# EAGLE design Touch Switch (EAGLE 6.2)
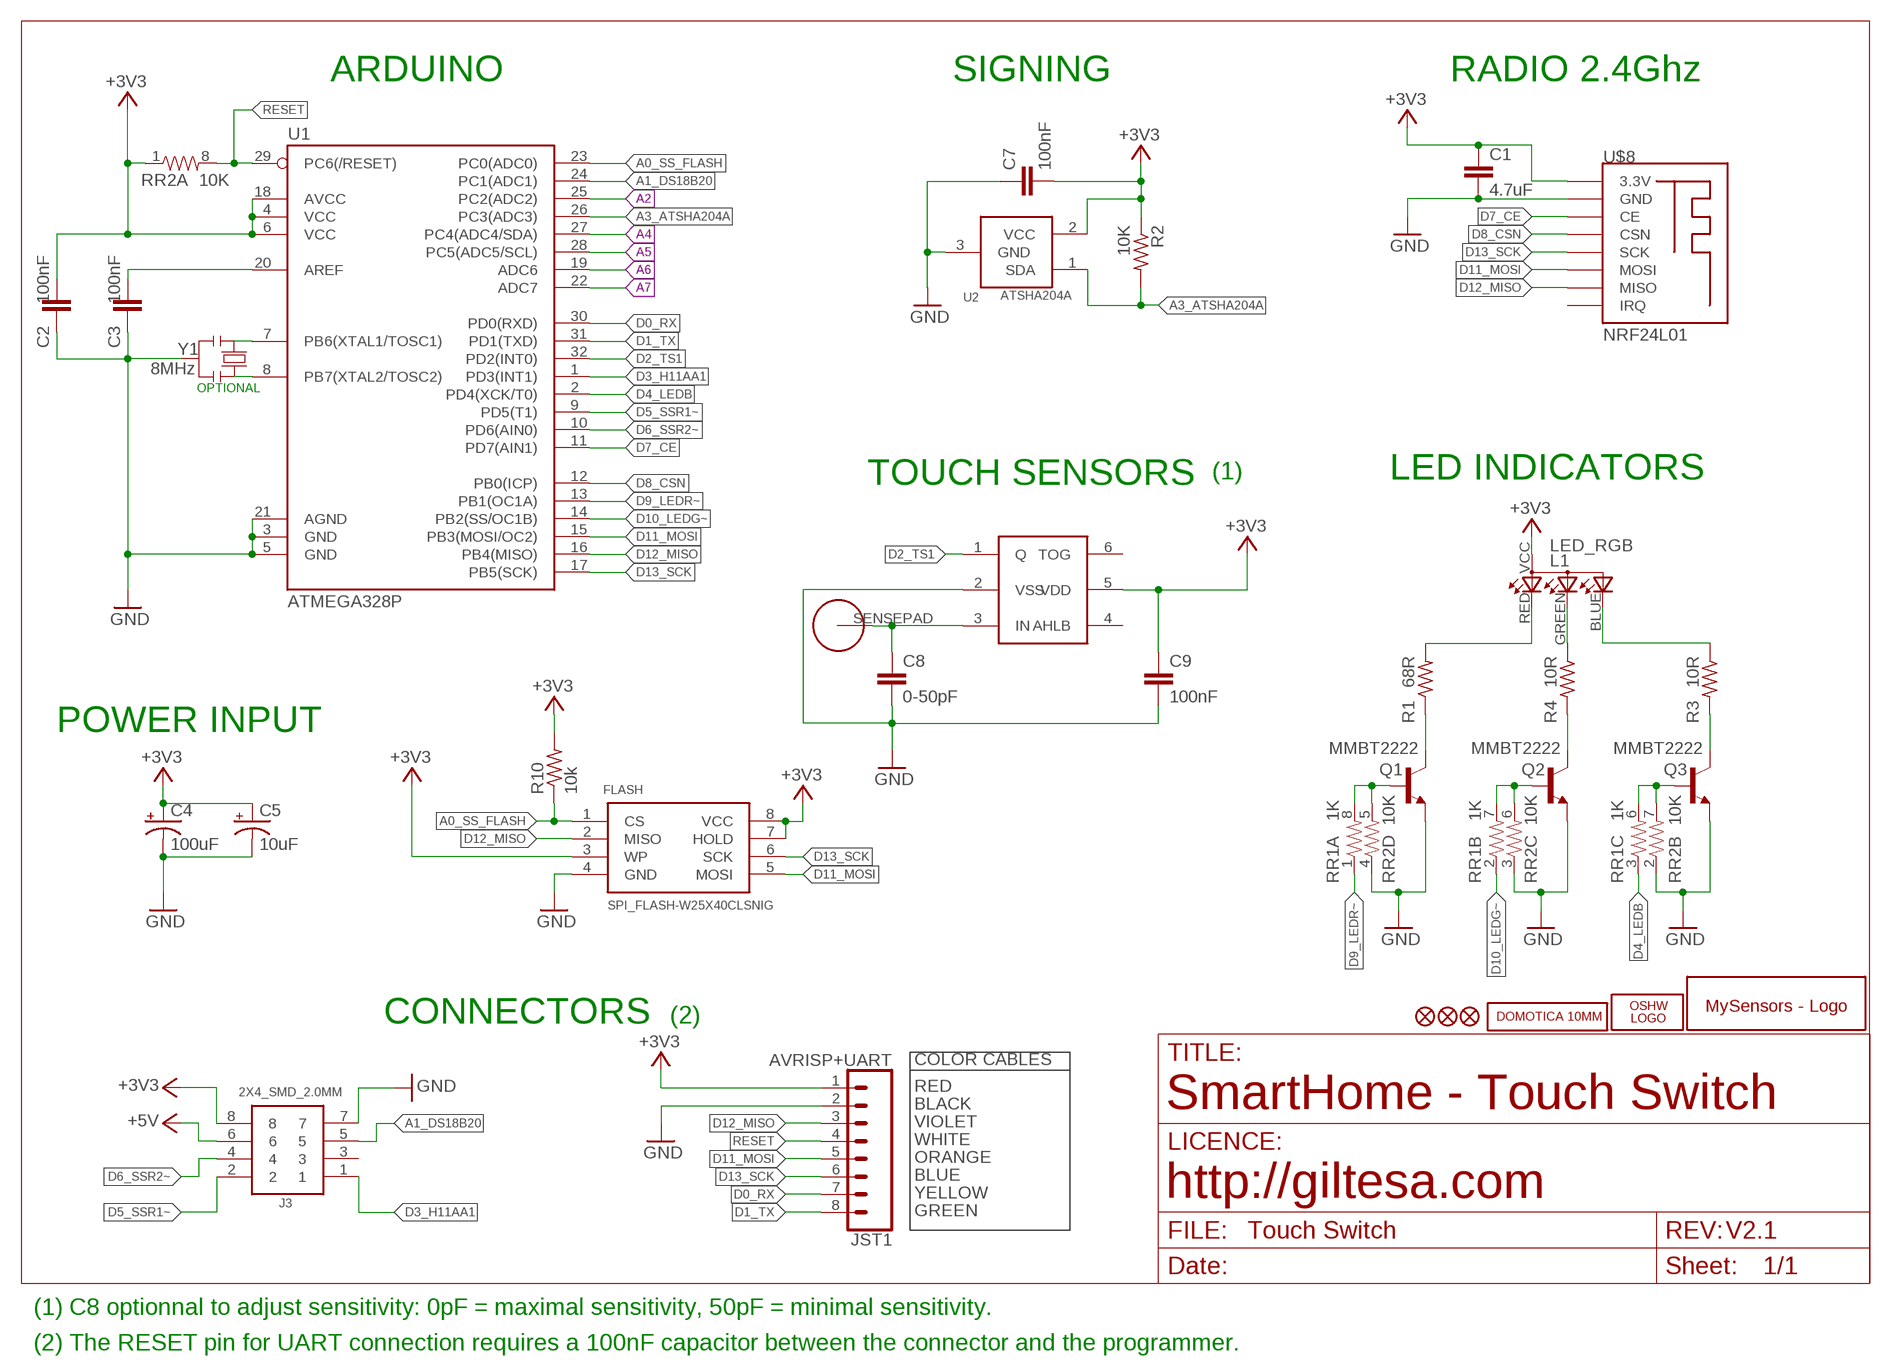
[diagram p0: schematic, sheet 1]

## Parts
C1  4.7uF  C1206  [C1206]
C2  100nF  C0603  [C0603]
C3  100nF  C0603  [C0603]
C4  100uF  10UF-16V-10%(TANT)  [EIA3216]
C5  10uF  10UF-16V-10%(TANT)  [EIA3216]
C7  100nF  C0603  [C0603]
C8  0-50pF  C0603  [C0603]
C9  100nF  C0603  [C0603]
FLASH  SPI_FLASH-W25X40CLSNIG  SPI_FLASH-X25XXSMD  [SO08]
J3  2X4_SMD_2.0MM  [2X4_SMD_2.0MM]
JST1  AVRISP+UART  JST-8-1MM-SMD  [JST-8-1MM-SMD]
L1  LED_RGB  LED_RGB_1206_SIDE  [LED_RGB_1206_SIDE]
LOGO1  OSHW_LOGO_FILLX0150-NT  [OSHW_FILLX150_NOTEXT]
Q1  MMBT2222  TRANSISTOR_NPNSOT23  [SOT23]
Q2  MMBT2222  TRANSISTOR_NPNSOT23  [SOT23]
Q3  MMBT2222  TRANSISTOR_NPNSOT23  [SOT23]
R1  68R  R0603  [R0603]
R2  10K  R0603  [R0603]
R3  10R  R0603  [R0603]
R4  10R  R0603  [R0603]
R10  10k  R0603  [R0603]
RR1  1K  RESISTOR-ARRAY0603-ARV  [0603-ARV]
RR2  10K  RESISTOR-ARRAY0603-ARV  [0603-ARV]
TTP1  TTP223  TTP223-BA6  [SOT-23-6]
U1  ATMEGA328P  ATMEGA328P_TQFP  [TQFP32-08]
U2  ATSHA204A  IC_ATSHA204A_CRYPT  [SOT23-3]
U$1  HTTM_SENSEPAD  [HTTM_SENSEPAD]
U$2  MYSENSORS  [MYSENSORS]
U$5  DOMOTICA-10MM  [DOMOTICA-10MM]
U$6  FIDUCIAL1X2  [FIDUCIAL-1X2]
U$7  FIDUCIAL1X2  [FIDUCIAL-1X2]
U$8  NRF24L01  NRF24L01_SMD  [NRF24L01_SMD]
U$14  FIDUCIAL1X2  [FIDUCIAL-1X2]
Y1  8MHz  RESONATORMU  [RESONATOR]

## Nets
+3V3: C1.1 C2.2 C4.A(+) C5.A(+) C7.2 C9.1 FLASH.3(WP) FLASH.7(HOLD) FLASH.8(VCC) J3.8 JST1.1 L1.VCC R2.1 R10.2 RR2.1 TTP1.5(VDD) U1.4(VCC) U1.6(VCC) U1.18(AVCC) U2.2(VCC) U$8.3.3V
+5V: J3.6
A0_SS_FLASH: FLASH.1(CS) R10.1 U1.23(PC0(ADC0))
A1_DS18B20: J3.5 U1.24(PC1(ADC1))
A2: U1.25(PC2(ADC2))
A3_ATSHA204A: R2.2 U1.26(PC3(ADC3)) U2.1(SDA)
A4: U1.27(PC4(ADC4/SDA))
A5: U1.28(PC5(ADC5/SCL))
A6: U1.19(ADC6)
A7: U1.22(ADC7)
D0_RX: JST1.7 U1.30(PD0(RXD))
D1_TX: JST1.8 U1.31(PD1(TXD))
D2_TS1: TTP1.1(Q) U1.32(PD2(INT0))
D3_H11AA1: J3.1 U1.1(PD3(INT1))
D4_LEDB: RR1.3 U1.2(PD4(XCK/T0))
D5_SSR1~: J3.2 U1.9(PD5(T1))
D6_SSR2~: J3.4 U1.10(PD6(AIN0))
D7_CE: U1.11(PD7(AIN1)) U$8.CE
D8_CSN: U1.12(PB0(ICP)) U$8.CSN
D9_LEDR~: RR1.1 U1.13(PB1(OC1A))
D10_LEDG~: RR1.2 U1.14(PB2(SS/OC1B))
D11_MOSI: FLASH.5(MOSI) JST1.5 U1.15(PB3(MOSI/OC2)) U$8.MOSI
D12_MISO: FLASH.2(MISO) JST1.3 U1.16(PB4(MISO)) U$8.MISO
D13_SCK: FLASH.6(SCK) JST1.6 U1.17(PB5(SCK)) U$8.SCK
GND: C1.2 C2.1 C3.1 C4.C(-) C5.C(-) C7.1 C8.2 C9.2 FLASH.4(GND) J3.7 JST1.2 Q1.2(E) Q2.2(E) Q3.2(E) RR2.2 RR2.3 RR2.4 TTP1.2(VSS) U1.3(GND) U1.5(GND) U1.21(AGND) U2.3(GND) U$8.GND Y1.2
N$1: Q1.3(C) R1.1
N$2: L1.GREEN R4.1
N$4: L1.RED R1.2
N$5: Q2.1(B) RR1.7 RR2.6
N$6: Q1.1(B) RR1.8 RR2.5
N$7: Q2.3(C) R4.2
N$8: Q3.3(C) R3.2
N$9: Q3.1(B) RR1.6 RR2.7
N$10: C8.1 TTP1.3(IN) U$1.SENSEPAD
N$11: L1.BLUE R3.1
N$29: U1.7(PB6(XTAL1/TOSC1)) Y1.1
N$30: U1.8(PB7(XTAL2/TOSC2)) Y1.3
N$33: C3.2 U1.20(AREF)
RESET: JST1.4 RR2.8 U1.29(PC6(/RESET))
Unconnected: J3.3 RR1.4 RR1.5 TTP1.4(AHLB) TTP1.6(TOG) U$8.IRQ

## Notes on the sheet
- ARDUINO | SIGNING | RADIO 2.4Ghz
- OPTIONAL
- TOUCH SENSORS | (1) | LED INDICATORS
- POWER INPUT
- CONNECTORS | (2)
- COLOR CABLES
- RED
- BLACK | SmartHome - Touch Switch
- VIOLET
- WHITE
- ORANGE
- BLUE
- YELLOW | http://giltesa.com
- GREEN
- V2.1
- (1) C8 optionnal to adjust sensitivity: 0pF = maximal sensitivity, 50pF = minimal sensitivity.
- (2) The RESET pin for UART connection requires a 100nF capacitor between the connector and the programmer.

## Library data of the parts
C1 = ,giltesa:C1206
C2 C3 C7-C9 = ,giltesa:C0603
C4 = SparkFun-Capacitors:10UF-16V-10%(TANT): CAP-00811; PROD_ID: CAP-00811; VALUE: 10uF
C5 = SparkFun-Capacitors:10UF-16V-10%(TANT): CAP-00811; PROD_ID: CAP-00811
FLASH = SparkFun-DigitalIC:SPI_FLASH-X25XX: 8pin SPI Flash series x25xx. Works with devices like W25X32 and BR25L32
J3 = ,giltesa:2X4_SMD_2.0MM
JST1 = ,giltesa:JST-8-1MM-SMD
L1 = ,giltesa:LED_RGB_1206_SIDE
LOGO1 = ohw-logo:OSHW_LOGO_FILL
Q1-Q3 = SparkFun:TRANSISTOR_NPN: Transistor NPN BJT configuration in SOT23 package. MMBT2222 is the common NPN we use. Double check BCE configuration again layout.
R1-R4 R10 = ,giltesa:R0603
RR1 RR2 = SparkFun-Passives:RESISTOR-ARRAY: Array Chip Resistor Source: RS Component / Phycomp
TTP1 = NCA_Sensors:TTP223-BA6: TTP223 touch sensor
U1 = SparkFun-DigitalIC:ATMEGA328P_TQFP; PROD_ID: IC-09069; VALUE: ATMEGA328P_TQFP
U2 = TD-MySensors:IC_ATSHA204A_CRYPT
U$1 = ,giltesa:HTTM_SENSEPAD
U$2 = ,giltesa_logos:MYSENSORS
U$5 = ,giltesa_logos:DOMOTICA-10MM
U$6 U$7 U$14 = SparkFun:FIDUCIAL: Fiducial Alignment Points
U$8 = ,giltesa:NRF24L01_SMD
Y1 = MySMD2:RESONATOR

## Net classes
1 POWER: width 0.457 mm, clearance 0.205 mm to class 0, clearance 0.254 mm

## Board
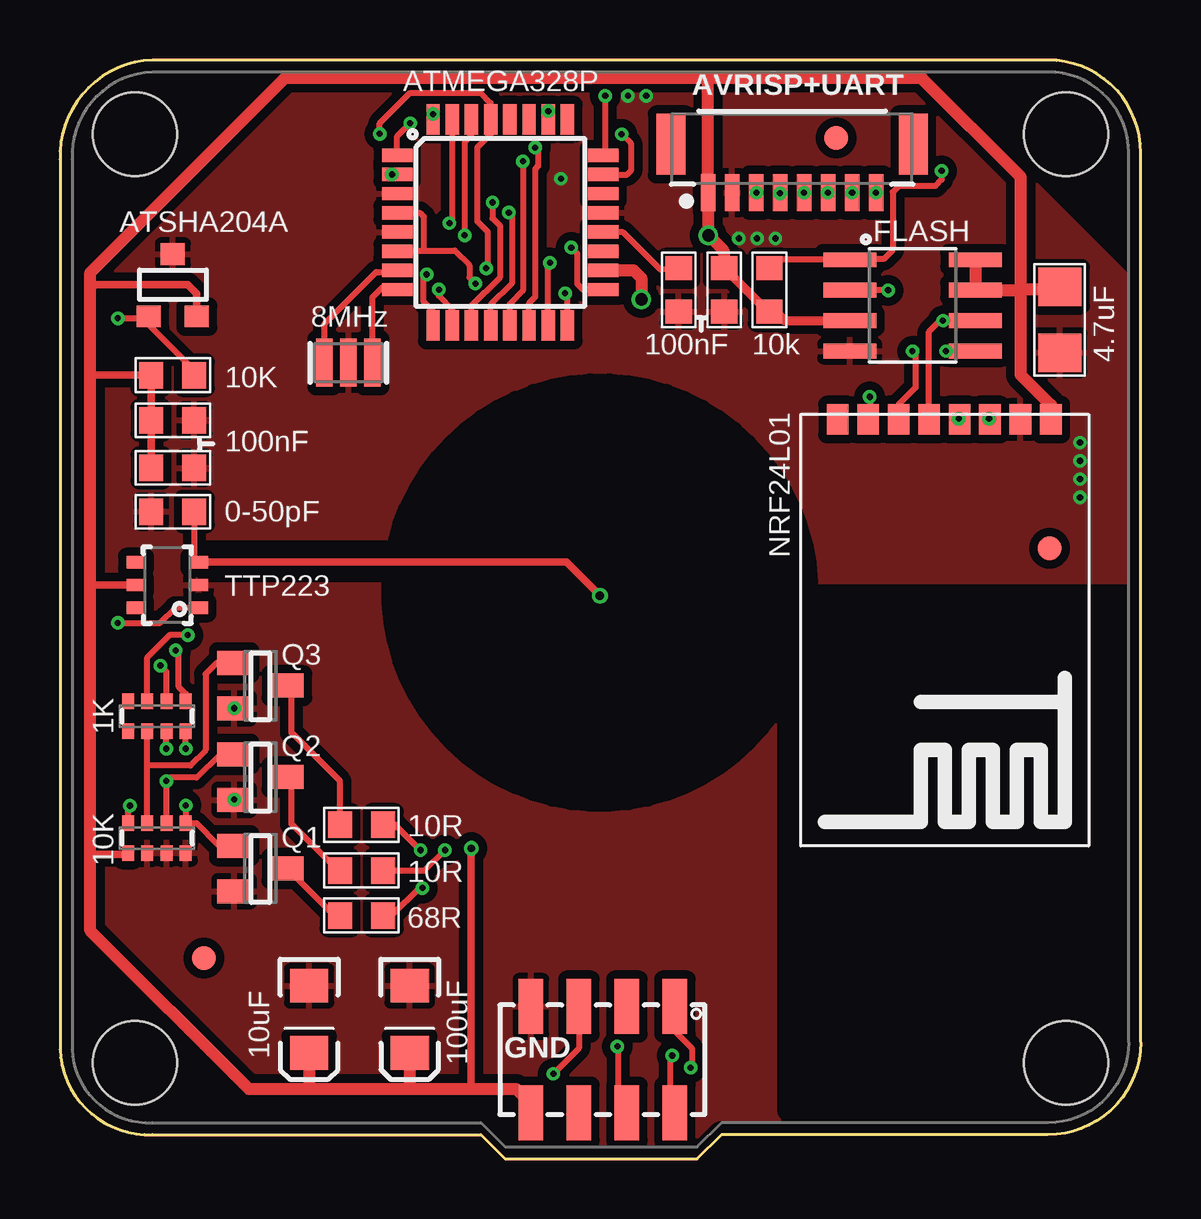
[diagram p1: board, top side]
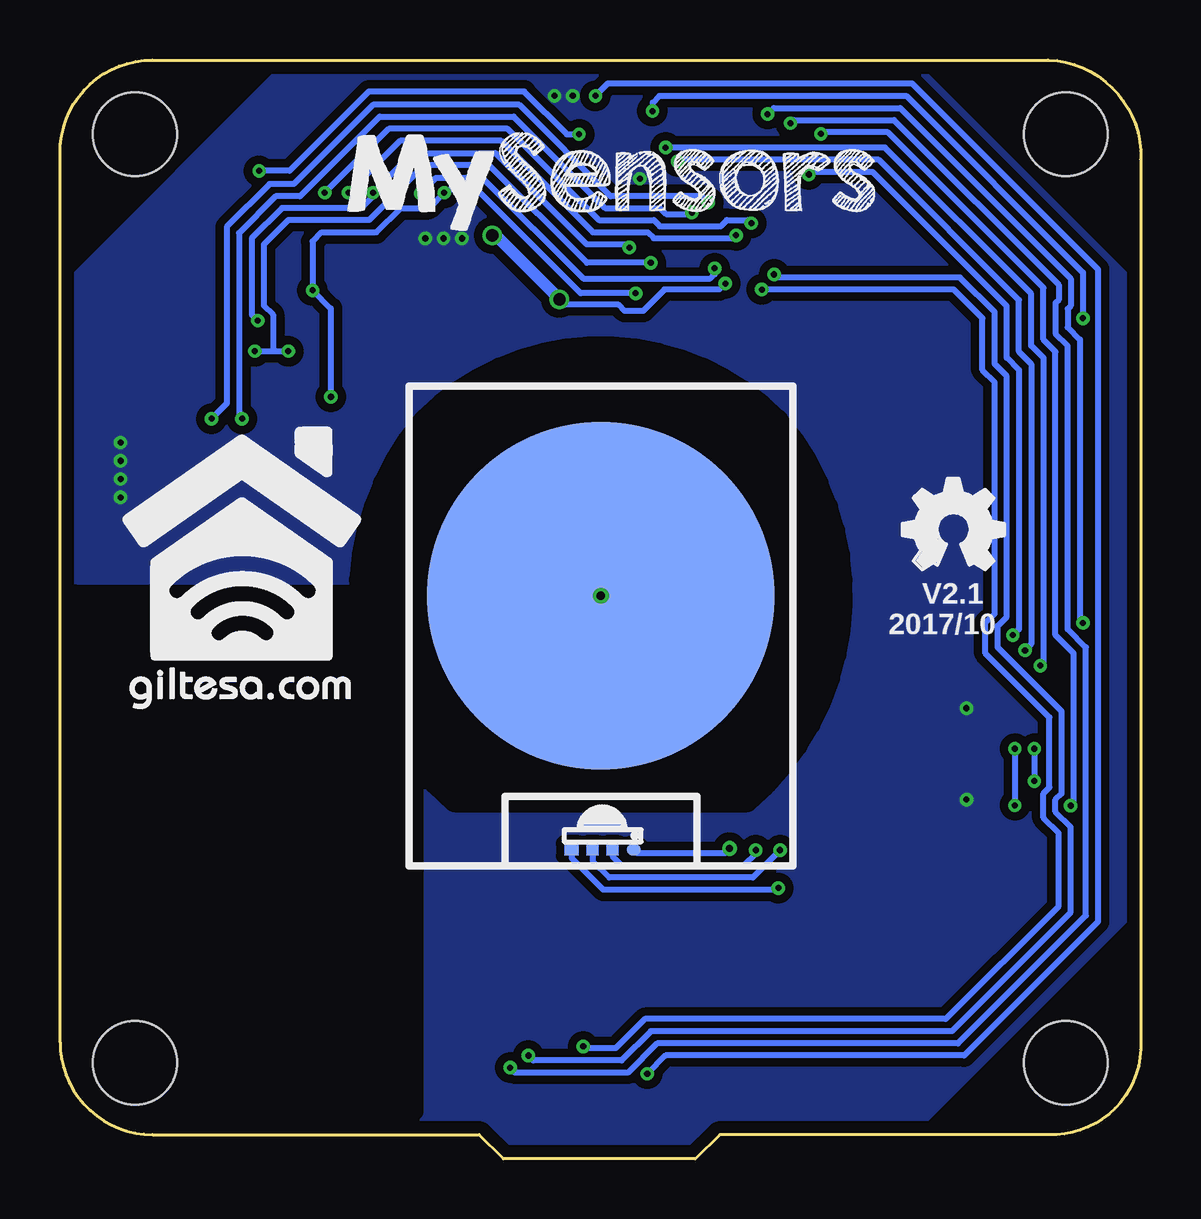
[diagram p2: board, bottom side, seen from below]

Size 45.05 x 45.81 mm. Coordinates in mm from the lower left corner, seen from the top.
Outline: 18.56,0 26.56,0 27.58,1.02 41.19,1.02 arc90 45.05,4.87 45.05,41.96 arc90 41.19,45.81 3.86,45.81 arc90 0,41.66 0,4.57 arc90 3.86,1.02 17.55,1.02 18.56,0
Copper layers (1*16): Top 0.035mm / dielectric 1.6mm / Bottom 0.035mm
Design rules: minimum track width 6mil, minimum drill 12mil, track to track 6mil, track to pad 6mil, pad to pad 6mil, via to via 8mil, smd to smd 0mil, copper to edge 20mil, drill to drill 10mil, minimum pad ring 6mil, minimum via ring 6mil, stop-mask expansion 0mil, vias tented up to drill 100mil, thermal gap 10mil
Holes 3.5 mm at 3.12,4.01 41.93,42.72 3.12,42.72 41.93,4.01
tRestrict: area 13.9,14.9 to 31.1,32.3; area 6.1,24.4 to 13.8,25.4; area 30.3,2 to 44.4,23.5
bRestrict: area 12.5,14.9 to 32.6,33.8; area 30.3,2 to 44.4,23.5

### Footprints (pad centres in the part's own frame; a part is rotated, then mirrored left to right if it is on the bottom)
C1206 = smd 1.6 x 1.8: 1 -1.362,-0.013; 2 1.387,-0.013
C0603 = smd 1 x 1.1: 1 -0.901,-0.038; 2 0.901,-0.038
EIA3216 = smd 1.4 x 1.6: A 1.4,0; C -1.4,0
SO08 = smd 0.61 x 2.21: 1 -1.905,-2.616; 2 -0.635,-2.616; 3 0.635,-2.616; 4 1.905,-2.616; 5 1.905,2.616; 6 0.635,2.616; 7 -0.635,2.616; 8 -1.905,2.616
2X4_SMD_2.0MM = smd 2.286 x 1.016: 1 -2.213,2.976; 2 2.212,2.976; 3 -2.213,0.976; 4 2.212,0.976; 5 -2.213,-1.024; 6 2.212,-1.024; 7 -2.213,-3.024; 8 2.212,-3.024
JST-8-1MM-SMD = smd 0.6 x 1.55: 1 -3.5,0; 2 -2.5,0; 3 -1.5,0; 4 -0.5,0; 5 0.5,0; 6 1.5,0; 7 2.5,0; 8 3.5,0 | smd 1.219 x 2.54: P$9 5.054,2.017; P$10 -5.054,2.017
LED_RGB_1206_SIDE = smd 0.5 x 0.5: BLUE -0.419,-0.83; GREEN 0.414,-0.83 | smd 0.6 x 0.5: RED -1.296,-0.83; VCC 1.295,-0.83
SOT23 = smd 1 x 1.4: 1 -0.95,-1.1; 2 0.95,-1.1; 3 0,1.1
R0603 = smd 1 x 1.1: 1 -0.901,0.013; 2 0.901,0.013
0603-ARV = smd 0.5 x 0.65: 1 -1.2,-0.625; 2 -0.4,-0.625; 3 0.4,-0.625; 4 1.2,-0.625; 5 1.2,0.625; 6 0.4,0.625; 7 -0.4,0.625; 8 -1.2,0.625
SOT-23-6 = smd 0.51 x 0.8: 1 0.955,-0.03; 2 1.905,-0.03; 3 2.855,-0.03; 4 2.855,2.57; 5 1.905,2.57; 6 0.955,2.57
TQFP32-08 = smd 1.27 x 0.559: 1 -4.293,2.8; 2 -4.293,2; 3 -4.293,1.2; 4 -4.293,0.4; 5 -4.293,-0.4; 6 -4.293,-1.2; 7 -4.293,-2; 8 -4.293,-2.8; 17 4.293,-2.8; 18 4.293,-2; 19 4.293,-1.2; 20 4.293,-0.4; 21 4.293,0.4; 22 4.293,1.2; 23 4.293,2; 24 4.293,2.8 | smd 0.559 x 1.27: 9 -2.8,-4.293; 10 -2,-4.293; 11 -1.2,-4.293; 12 -0.4,-4.293; 13 0.4,-4.293; 14 1.2,-4.293; 15 2,-4.293; 16 2.8,-4.293; 25 2.8,4.293; 26 2,4.293; 27 1.2,4.293; 28 0.4,4.293; 29 -0.4,4.293; 30 -1.2,4.293; 31 -2,4.293; 32 -2.8,4.293
SOT23-3 = smd 1 x 0.9: 1 -1,-1.3; 2 1,-1.3; 3 0,1.3
HTTM_SENSEPAD = smd 14.5 x 14.5: SENSEPAD -0.001,0.001
FIDUCIAL-1X2 = smd 1 x 1: 1 0,0
NRF24L01_SMD = smd 0.9 x 1.27: 3.3V 1.575,0.203; CE 4.115,0.203; CSN 5.385,0.203; GND 2.845,0.203; IRQ 10.465,0.203; MISO 9.195,0.203; MOSI 7.925,0.203; SCK 6.655,0.203
RESONATOR = smd 0.7 x 2: 1 -1,0; 2 0,0; 3 1,0

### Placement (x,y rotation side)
C1  41.69,35 270 top
C2  27.65,36.23 90 top
C3  25.75,36.23 90 top
C4  14.58,5.83 270 top
C5  10.38,5.83 270 top
C7  4.7,30.75 180 top
C8  4.7,26.94 180 top
C9  4.7,28.85 0 top
FLASH  35.54,35.58 270 top
J3  22.66,4.15 270 top
JST1  30.52,40.28 0 top
L1  22.43,13.73 0 bottom
LOGO1  9.93,24.56 0 bottom
Q1  8.36,12.11 270 top
Q2  8.36,15.92 270 top
Q3  8.36,19.73 270 top
R1  12.57,10.14 0 top
R2  4.7,32.66 0 top
R3  12.57,13.95 180 top
R4  12.57,12.04 180 top
R10  29.56,36.23 270 top
RR1  4.04,18.46 180 top
RR2  4.04,13.38 0 top
TTP1  5.74,22.02 90 top
U1  18.35,39.04 0 top
U2  4.7,36.42 0 top
U$1  22.5,23.48 0 bottom
U$2  33.05,38.5 0 bottom
U$5  42.46,18.69 0 bottom
U$6  41.25,25.45 0 top
U$7  32.36,42.57 0 top
U$8  42.88,31.03 180 top
U$14  6,8.38 0 top
Y1  12.02,33.19 0 top

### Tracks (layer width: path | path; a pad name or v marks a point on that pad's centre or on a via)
+3V3  (via drill 0.25, 0.3, 0.51)
  Top 0.254: R10.2 29.35,35.38 | U1.6 14.09,37.87 15.16,37.87 | v17.32,36.49 17.06,36.75 17.06,37.26 16.45,37.87 15.16,37.87 | U1.4 15.01,39.44 15.16,39.29 15.16,37.87
  Top 0.305: RR2.1 2.78,12.7 1.27,12.7 | TTP1.5 1.34,23.93 1.27,24 | C9.1 C7.2 R2.1 1.35,32.67 1.27,32.76 | U2.2 5.7,36.07 5.33,36.44 1.39,36.44 1.27,36.32 | v17.14,12.95 17.14,2.99 17.06,2.92
  Top 0.381: 29.77,35.38 30.2,34.95 FLASH.3 | 29.35,35.38 29.35,35.47 C2.2
  Top 0.508: v24.23,35.84 24.23,36.72 23.92,37.04 U1.18 | 27.02,38.64 v27.03,38.5 | v27.03,38.5 27.65,37.88 C2.2 | 29.77,35.38 R10.2 | 26.84,45.08 9.39,45.08 1.27,36.95 1.27,36.32 1.27,32.76 1.27,24 1.27,12.7 1.27,9.52 7.87,2.92 10.33,2.92 | 26.84,45.08 35.91,45.08 40.05,40.94 40.05,36.24 | 10.33,2.92 14.52,2.92 | 14.52,2.92 17.06,2.92 19.02,2.92 19.48,2.46 19.48,2.09 J3.8 | C5.A 10.38,2.97 10.33,2.92 | C4.A 14.58,2.97 14.52,2.92 | 26.84,45.08 27.02,45.03 JST1.1 v27.02,38.51 v27.03,38.5 | U$8.3.3V 41.3,31.43 40.05,32.69 40.05,36.24 | 40.05,36.24 40.03,36.22 FLASH.7 FLASH.8 | C1.1 41.68,36.34 41.57,36.24 40.05,36.24
  Bottom 0.254: v17.14,12.95 17.12,12.95 17.32,12.75 20.98,12.75 L1.VCC | v17.32,36.49 17.57,36.24 19.86,36.24 20.75,35.35 21.51,35.35 21.76,35.61 24,35.61 v24.23,35.84
  Bottom 0.508: v24.23,35.84 26.9,38.5 v27.03,38.5
A0_SS_FLASH  (via drill 0.25)
  Top 0.254: R10.1 arc-90 29.97,37.49 FLASH.1 32.95,37.51 34.34,37.51 34.72,37.89 34.72,40.3 34.97,40.56 36.49,40.56 36.75,40.81 v36.75,41.19 | U1.23 23.64,41.04 23.8,41.19 23.8,42.34 v23.41,42.72
  Bottom 0.254: v36.75,41.19 35.48,41.19 32.18,44.5 25.7,44.5 23.92,42.72 v23.41,42.72
A1_DS18B20  (via drill 0.25)
  Top 0.254: v22.73,44.32 22.73,41.92 U1.24 | 21.46,7.08 J3.5 21.63,4.61 v20.57,3.55
  Bottom 0.254: v22.73,44.32 22.22,44.83 9.52,44.83 1.77,37.08 1.77,9.9 7.36,4.31 19.81,4.31 v20.57,3.55
A3_ATSHA204A  (via drill 0.25)
  Top 0.254: R2.2 5.31,32.9 5.31,33.17 3.7,34.78 U2.1 3.63,35.05 v2.41,35.05 | U1.26 20.35,43.65 v20.35,43.68
  Bottom 0.254: v20.35,43.68 20.34,44.04 20.06,44.32 9.78,44.32 2.41,36.95 v2.41,35.05
D0_RX  (via drill 0.25)
  Top 0.254: JST1.7 32.89,40.41 JST1.7 | v16.87,38.5 16.89,38.52 16.89,42.41 17.14,42.67 U1.30
  Bottom 0.254: v16.87,38.5 16.99,38.38 20.3,38.38 20.55,38.63 22.84,38.63 26.65,42.44 30.86,42.44 JST1.7
  other vias: 33.02,40.28
D1_TX  (via drill 0.25)
  Top 0.254: U1.31 16.35,39.13 v16.23,39.01 | v34.01,40.28 33.89,40.41 JST1.8
  Bottom 0.254: v16.23,39.01 16.36,39.14 17.25,39.14 17.5,38.88 20.04,38.88 20.3,39.14 22.58,39.14 26.39,42.95 31.35,42.95 v34.01,40.28
D2_TS1  (via drill 0.25)
  Top 0.254: U1.32 15.55,43.37 v15.55,43.56 | v2.41,22.35 4.19,22.35 4.82,22.98 TTP1.1
  Bottom 0.254: v15.55,43.56 15.3,43.81 10.03,43.81 2.92,36.7 2.92,35.55 3.04,35.43 3.04,34.67 2.54,34.16 2.54,22.47 v2.41,22.35
D3_H11AA1  (via drill 0.25)
  Top 0.254: U1.1 14.06,42.63 v14.6,43.17 | J3.1 25.52,7.15 25.52,5.43 26.34,4.62 26.34,3.86 v26.29,3.81
  Bottom 0.254: v14.6,43.17 14.47,43.3 10.28,43.3 3.42,36.44 3.42,35.81 3.55,35.68 3.55,34.41 3.04,33.9 3.04,22.09 2.28,21.33 2.28,10.15 7.62,4.82 20.16,4.82 21.38,3.6 26.08,3.6 v26.29,3.81
D4_LEDB  (via drill 0.25)
  Top 0.254: U1.2 13.74,41.04 v13.84,41.04 | v5.33,21.84 4.57,21.84 3.64,20.91 RR1.3
  Bottom 0.254: v13.84,41.04 13.74,41.14 11.17,41.14 5.58,35.55 5.58,33.4 5.08,32.89 5.08,22.09 v5.33,21.84
D5_SSR1~  (via drill 0.25)
  Top 0.254: J3.2 25.63,2.15 25.45,2.33 25.45,4.24 v25.52,4.31 | U1.9 15.54,34.76 15.54,35.35 15.16,35.73 15.16,36.75 v15.29,36.88
  Bottom 0.254: v25.52,4.31 25.32,4.11 21.64,4.11 20.42,5.33 7.87,5.33 2.92,10.28 2.92,13.84 3.55,14.47 3.55,14.98 3.3,15.23 3.3,18.66 5.96,21.33 5.96,22.22 5.58,22.6 5.58,32.63 6.09,33.14 6.09,35.3 7.54,36.75 15.16,36.75 v15.29,36.88
D6_SSR2~  (via drill 0.25)
  Top 0.254: J3.4 23.63,1.99 23.29,2.33 23.29,4.62 v23.24,4.69 | v15.79,36.24 15.79,35.99 16.35,35.43 U1.10
  Bottom 0.254: v23.24,4.69 23.29,4.62 21.89,4.62 20.67,5.84 8.12,5.84 3.42,10.54 3.42,13.58 4.06,14.22 4.06,15.23 3.81,15.49 3.81,18.41 6.47,21.08 6.47,22.35 6.09,22.73 6.09,32.38 6.6,32.89 6.6,35.05 7.79,36.24 v15.79,36.24
D7_CE  (via drill 0.25)
  Top 0.254: U1.11 17.14,35.55 18.33,36.75 18.33,38.91 18.03,39.21 v18.03,39.87 | v38.73,30.86 U$8.CE
  Bottom 0.254: v38.73,30.86 38.1,31.49 38.1,38.86 36.32,40.63 35.3,40.63 32,43.94 25.9,43.94 22.09,40.13 18.28,40.13 v18.03,39.87
D8_CSN  (via drill 0.25)
  Top 0.254: v37.46,30.86 U$8.CSN | U1.12 17.95,35.61 18.84,36.49 18.84,39.29 18.71,39.42 v18.71,39.45
  Bottom 0.254: v37.46,30.86 37.59,30.98 37.59,38.6 36.06,40.13 35.05,40.13 34.9,40.27 34.9,40.28 31.73,43.45 26.14,43.45 22.33,39.65 20.04,39.65 19.79,39.39 18.77,39.39 v18.71,39.45
D9_LEDR~  (via drill 0.25)
  Top 0.254: U1.13 18.75,35.64 19.3,36.19 v19.3,41.59 | RR1.1 5.24,19.39 4.95,19.68 4.95,21.08 v4.82,21.2
  Bottom 0.254: v4.82,21.2 4.57,21.46 4.57,33.14 5.08,33.65 5.08,35.81 10.92,41.65 19.24,41.65 v19.3,41.59
D10_LEDG~  (via drill 0.25)
  Top 0.254: v19.81,42.16 19.94,42.03 19.94,41.4 19.81,41.27 19.81,35.94 19.55,35.68 U1.14 | RR1.2 4.44,20.32 v4.19,20.57
  Bottom 0.254: v19.81,42.16 10.66,42.16 4.57,36.06 4.57,33.9 4.06,33.4 4.06,20.7 v4.19,20.57
D11_MOSI  (via drill 0.25)
  Top 0.254: FLASH.5 v36.93,33.68 | v35.54,33.68 35.66,33.55 35.66,32.15 34.95,31.44 U$8.MOSI | U1.15 20.35,37.29 v20.42,37.36 | JST1.5 30.89,40.41 JST1.5
  Bottom 0.254: v36.93,33.68 36.17,33.68 | 36.17,33.68 v35.54,33.68 | v20.42,37.36 23.09,37.36 27.15,41.42 29.87,41.42 JST1.5 32.16,39.14 35.54,39.14 36.55,38.12 36.55,35.58 36.17,35.2 36.17,33.68
  other vias: 31.02,40.28
D12_MISO  (via drill 0.25)
  Top 0.254: U1.16 21.15,35.99 v21.06,36.09 | v29.03,40.28 28.89,40.41 JST1.3 | v34.52,36.22 FLASH.2 | v33.76,31.77 33.76,30.91 U$8.MISO
  Bottom 0.254: v21.06,36.09 23.34,36.09 27.66,40.41 28.8,40.41 v29.03,40.28 29.67,39.65 30.84,39.65 31.85,38.63 34.14,38.63 34.52,38.25 v34.52,36.22 33.76,35.45 v33.76,31.77
D13_SCK  (via drill 0.25)
  Top 0.254: U$8.SCK 36.22,34.49 36.68,34.95 v36.81,34.95 FLASH.6 | U1.17 21.8,36.24 21.57,36.47 21.57,37.74 v21.31,37.99 | v32.01,40.28 31.89,40.41 JST1.6
  Bottom 0.254: v21.31,37.99 21.44,38.12 23.09,38.12 26.9,41.93 30.36,41.93 v32.01,40.28 31.98,40.15 32.49,39.65 35.79,39.65 37.06,38.38 37.06,35.2 v36.81,34.95
GND  (via drill 0.25)
  other vias: 42.52,29.87 42.52,29.1 42.52,28.34 42.52,27.58 28.3,38.37 29.06,38.37 29.82,38.37 7.27,18.79 7.27,14.98 20.88,40.86 23.67,44.32 24.44,44.32
  pour Bottom (isolate 0.356): 9.83,46.15 35.22,46.15 45.26,36.11 45.26,10.71 35.22,0.68 27.73,0.68 26.72,-0.33 18.33,-0.33 17.32,0.68 9.83,0.68 -0.21,10.71 -0.21,36.11
  pour Top (isolate 0.356): 9.83,46.15 35.22,46.15 45.26,36.11 45.26,10.71 35.22,0.68 27.73,0.68 26.72,-0.33 18.33,-0.33 17.32,0.68 9.83,0.68 -0.21,10.71 -0.21,36.11
N$1
  Top 0.254: R1.1 11.42,10.15 Q1.3
N$2  (via drill 0.25)
  Top 0.254: R4.1 15.2,12.03 v16.05,12.87
  Bottom 0.254: v16.05,12.87 16.05,12.75 16.56,12.24 21.64,12.24 22.02,12.62 L1.GREEN
N$4  (via drill 0.25)
  Top 0.254: R1.2 13.83,10.15 14.98,11.3 v15.11,11.3
  Bottom 0.254: v15.11,11.3 15.19,11.22 22.4,11.22 23.73,12.55 L1.RED
N$5  (via drill 0.25)
  Top 0.254: Q2.1 6.67,16.87 5.69,15.9 4.57,15.9 v4.43,15.76 RR2.6 4.48,14.05 | v4.43,17.1 RR1.7
  Bottom 0.254: v4.43,17.1 v4.43,15.76
N$6  (via drill 0.25)
  Top 0.254: Q1.1 6.62,13.06 5.69,13.99 5.13,13.99 RR2.5 5.25,13.89 v5.25,14.74 | v5.25,17.1 RR1.8
  Bottom 0.254: v5.25,17.1 v5.25,14.74
N$7
  Top 0.254: 11.58,12.03 9.65,13.96 9.65,15.73 Q2.3
  Top 0.406: R4.2 11.58,12.03
N$8
  Top 0.254: R3.2 11.67,15.76 9.65,17.77 9.65,19.54 Q3.3
N$9
  Top 0.254: RR2.7 3.64,16.4 | 3.64,16.4 RR1.6 | Q3.1 6.54,20.68 6.07,20.21 6.07,17.04 5.44,16.4 3.64,16.4
N$10  (via drill 0.36)
  Top 0.254: 5.55,24.88 TTP1.3 5.6,25.05 C8.1
  Top 0.305: TTP1.3 21.11,24.88 v22.5,23.48
  Bottom 0.127: U$1.SENSEPAD v22.5,23.48 | v22.5,23.48
  Bottom 0.305: v22.5,23.48 22.41,24.28
  Bottom 0.406: 22.46,24.18 v22.5,23.48
N$11  (via drill 0.25)
  Top 0.254: R3.1 13.97,13.93 v15.03,12.87
  Bottom 0.254: v15.03,12.87 16.18,11.73 22.14,11.73 22.85,12.44 L1.BLUE
N$29
  Top 0.254: Y1.1 11.02,34.81 13.18,36.98 14.14,36.98 | 14.14,36.98 14.45,36.98 | U1.7 14.12,37.1 14.12,36.99 14.14,36.98
N$30
  Top 0.254: Y1.3 13.02,35.93 13.44,36.34 13.96,36.34 U1.8
N$33
  Top 0.254: C3.2 25.02,37.08 23.47,38.63 U1.20
RESET  (via drill 0.25)
  Top 0.254: v30.02,40.25 JST1.4 | RR2.8 2.84,14.65 v2.92,14.73 | v13.33,42.73 13.33,43.17 14.6,44.45 17.52,44.45 17.95,44.01 U1.29 17.95,42.72 17.39,42.16 17.39,39.09 17.83,38.65 17.83,37.19 v17.76,37.13
  Bottom 0.254: v30.02,40.25 29.38,40.89 27.43,40.89 23.24,36.7 17.94,36.7 17.76,36.88 v17.76,37.13 | v2.92,14.73 2.79,14.85 2.79,21.08 3.55,21.84 3.55,33.65 4.06,34.16 4.06,36.32 10.54,42.79 13.27,42.79 v13.33,42.73

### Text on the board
tPlace: GND
bPlace: V2.1 | 2017/10

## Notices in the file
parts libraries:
SparkFun-DigitalIC: Licensing: Creative Commons ShareAlike 4.0 International - https://creativecommons.org/licenses/by-sa/4.0
